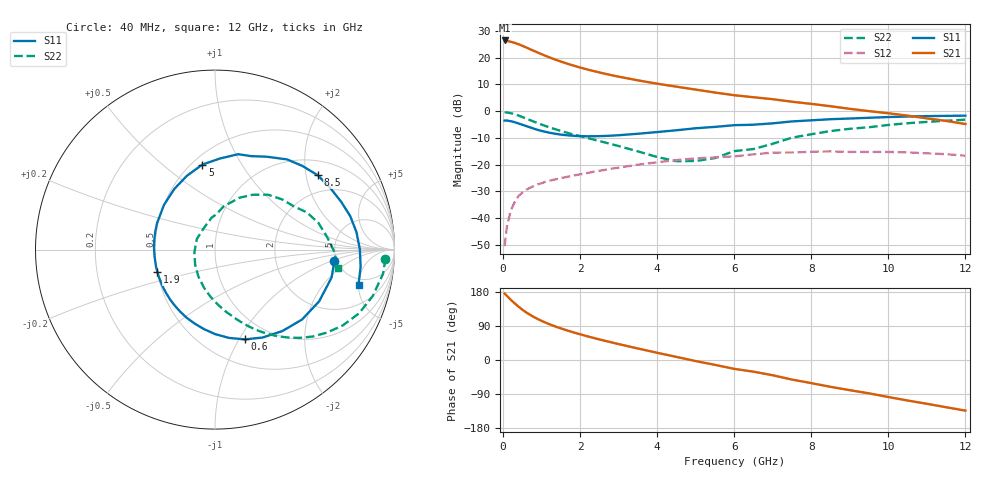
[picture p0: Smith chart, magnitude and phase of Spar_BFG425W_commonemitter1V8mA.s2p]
! Filename: 18bfg425.001
! BFG425W Field C1
! V1=8.472E-001V,V2=1.000E+000V, I1=1.149E-004A, I2=7.990E-003A
# GHz  S  MA  R 50
!  S11  S21  S12  S22
!Freq(GHz)  Mag  Ang  Mag  Ang  Mag  Ang  Mag  Ang
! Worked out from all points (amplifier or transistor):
!   44 points, 40 MHz to 12 GHz, reference 50 ohm
!   highest |S21| = 26.4 dB at 40 MHz (marker M1)
!   |S21| within 3 dB of that: start of sweep to 659.5 MHz
!   unconditionally stable (mu >= 1): 1.979 GHz to end of sweep
!   at 700 MHz: K = 0.48, MSG = 25.9 dB, |S12| = -28.6 dB
!   at 2.4 GHz: K = 1.09, MAG = 16.8 dB, |S12| = -22.5 dB
!   at 12 GHz: K = 1.42, MAG = 2.1 dB, |S12| = -16.7 dB
!   S11 on the Smith chart (normalised r, x): 40 MHz: 4.77, -1.09; 600 MHz: 0.76, -1.06; 1.9 GHz: 0.50, -0.14; 5 GHz: 0.56, +0.69; 8.5 GHz: 1.42, +2.34; 12 GHz: 4.14, -4.99
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0.04  0.668 -5.4  20.94 175.4  0.003 82.8  0.951 -3.0
0.1  0.668 -13.4  20.5 169.2  0.007 82.6  0.946 -8.2
0.2  0.648 -26.4  19.79 158.9  0.014 76.0  0.916 -16.4
0.3  0.622 -38.8  18.9 149.7  0.02 70.0  0.877 -23.9
0.4  0.589 -50.4  17.81 140.9  0.026 64.7  0.828 -30.7
0.5  0.557 -61.6  16.67 132.8  0.03 60.1  0.777 -36.5
0.6  0.527 -71.6  15.49 125.7  0.034 56.5  0.728 -41.7
0.8  0.471 -89.9  13.37 113.4  0.04 50.5  0.636 -50.4
0.9  0.447 -98.0  12.45 108.1  0.043 48.3  0.597 -54.0
1.1  0.411 -112.7  10.82 98.7  0.048 44.9  0.529 -60.3
1.3  0.384 -125.8  9.508 90.6  0.052 42.2  0.473 -65.7
1.5  0.365 -137.8  8.45 83.4  0.056 40.2  0.427 -70.4
1.9  0.344 -159.0  6.855 70.7  0.064 36.6  0.356 -79.3
2.2  0.339 -172.9  5.978 62.2  0.07 34.0  0.313 -85.9
3  0.355 155.3  4.409 42.0  0.088 26.2  0.223 -105.5
3.5  0.378 138.7  3.764 30.3  0.1 20.3  0.177 -121.4
4.5  0.44 110.9  2.865 8.2  0.122 7.0  0.116 -172.3
5  0.479 98.4  2.528 -2.8  0.131 -1.0  0.117 149.8
6.5  0.558 69.0  1.82 -30.8  0.156 -19.0  0.196 88.1
8.5  0.707 35.8  1.236 -70.9  0.177 -54.3  0.425 46.1
10.5  0.794 7.1  0.824 -106.9  0.17 -87.7  0.595 14.5
12  0.823 -13.7  0.575 -133.6  0.147 -116.1  0.694 -8.3
